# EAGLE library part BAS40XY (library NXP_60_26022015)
General-purpose Schottky diodes General-purpose Schottky diodes in small Surface-Mounted Device (SMD) plastic packages. AAL Eindhoven MK
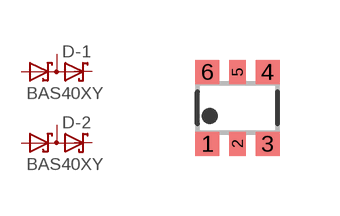
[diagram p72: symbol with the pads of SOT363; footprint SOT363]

Designator prefix D; gates -1=DIODE_SDD_AKAK -2=DIODE_SDD_AKAK

## BAS40XY  [SOT363]
1  -1:A1  pas
2  -1:K2  pas
3  -2:K1A2  pas
4  -2:A1  pas
5  -2:K2  pas
6  -1:K1A2  pas

## Footprint SOT363 (pad centres in mm)
SOT363 Plastic surface-mounted package; 6 leads JEDEC: -- IEC: -- JEITA: SC-88
smd 0.6 x 0.6: 1 -0.75,-0.9; 3 0.75,-0.9; 4 0.75,0.9; 6 -0.75,0.9
smd 0.4 x 0.6: 2 0,-0.9; 5 0,0.9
